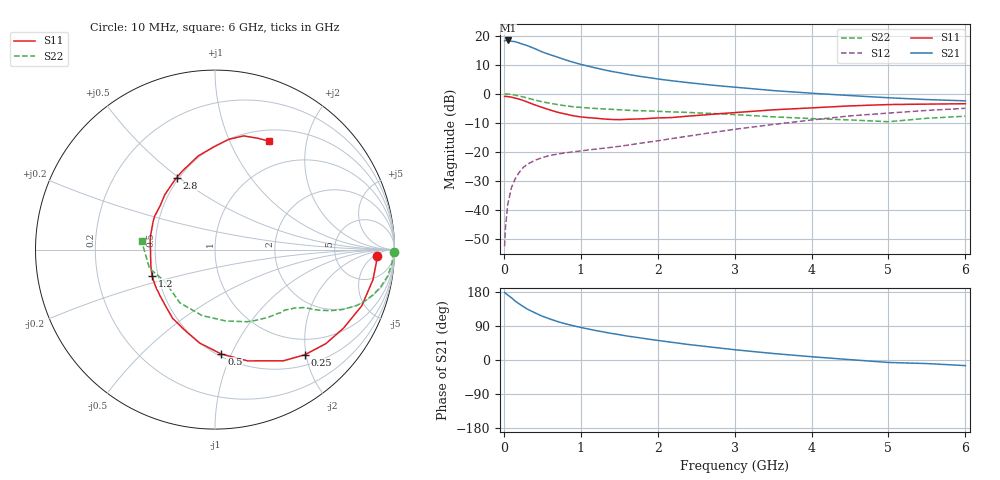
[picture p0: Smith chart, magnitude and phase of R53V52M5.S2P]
! SIEMENS Small Signal Semiconductors
! BFR183
! Si NPN RF Bipolar Junction Transistor in SOT23
! VCE = 3.5 V  IC = 2.5 mA
! Common Emitter S-Parameters:  May  1996
# GHz  S  MA  R  50
!  f  S11  S21  S12  S22
! GHz  MAG  ANG  MAG  ANG  MAG  ANG  MAG  ANG
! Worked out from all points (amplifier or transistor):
!   36 points, 10 MHz to 6 GHz, reference 50 ohm
!   highest |S21| = 18.3 dB at 50 MHz (marker M1)
!   |S21| within 3 dB of that: start of sweep to 418.7 MHz
!   unconditionally stable (mu >= 1): 1.318 GHz to 2.792 GHz
!   at 250 MHz: K = 0.26, MSG = 21.2 dB, |S12| = -25.4 dB
!   at 1.4 GHz: K = 1.03, MAG = 11.9 dB, |S12| = -18.4 dB
!   at 6 GHz: K = 0.89, MSG = 1.3 dB, |S12| = -5.0 dB
!   S11 on the Smith chart (normalised r, x): 10 MHz: 17, -6; 250 MHz: 0.69, -1.98; 500 MHz: 0.52, -0.92; 1.2 GHz: 0.46, -0.16; 2.8 GHz: 0.48, +0.49; 6 GHz: 0.64, +1.42
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0.01  0.9031 -2.2  8.119 178.6  0.0024 89.3  0.9957 -0.8
0.02  0.902 -4.4  8.263 176.6  0.0048 87.8  0.9911 -1.8
0.05  0.896 -10.8  8.265 171.7  0.0124 85.8  0.9891 -4.4
0.15  0.8393 -31.4  7.861 155.1  0.0351 72.6  0.9469 -12.6
0.2  0.81 -40.3  7.479 148.2  0.0446 68.9  0.9156 -16.0
0.25  0.7705 -49.5  7.086 141.4  0.0537 64.1  0.8836 -18.9
0.3  0.7274 -58.4  6.772 134.9  0.0608 60.6  0.8494 -21.5
0.4  0.6464 -73.6  6.002 124.9  0.0716 55.0  0.7828 -25.3
0.5  0.5831 -86.5  5.238 115.6  0.0802 51.1  0.729 -27.8
0.6  0.5277 -99.3  4.711 108.1  0.0871 48.3  0.6876 -29.5
0.7  0.4809 -110.2  4.263 101.4  0.0922 47.0  0.6528 -30.9
0.8  0.4497 -121.7  3.84 95.6  0.0964 46.0  0.6222 -31.9
0.9  0.4199 -130.5  3.495 90.5  0.1005 46.1  0.5993 -32.7
1.1  0.3889 -149.1  2.979 81.7  0.1086 46.4  0.5708 -34.7
1.2  0.3795 -157.6  2.773 77.6  0.1121 46.9  0.5585 -35.6
1.6  0.364 173.1  2.172 63.3  0.1305 50.4  0.5222 -39.8
2.2  0.3916 141.1  1.666 46.3  0.1713 54.4  0.4884 -48.7
2.8  0.4549 118.1  1.371 31.7  0.2242 54.1  0.4526 -61.0
3.5  0.5303 100.1  1.137 17.2  0.2967 49.0  0.4021 -81.4
4.5  0.6196 82.8  0.933 1.0  0.4169 37.6  0.3554 -123.4
5.5  0.6648 68.9  0.796 -9.4  0.5177 23.5  0.3795 -164.0
6  0.6752 63.5  0.757 -14.8  0.5628 14.6  0.412 173.3
